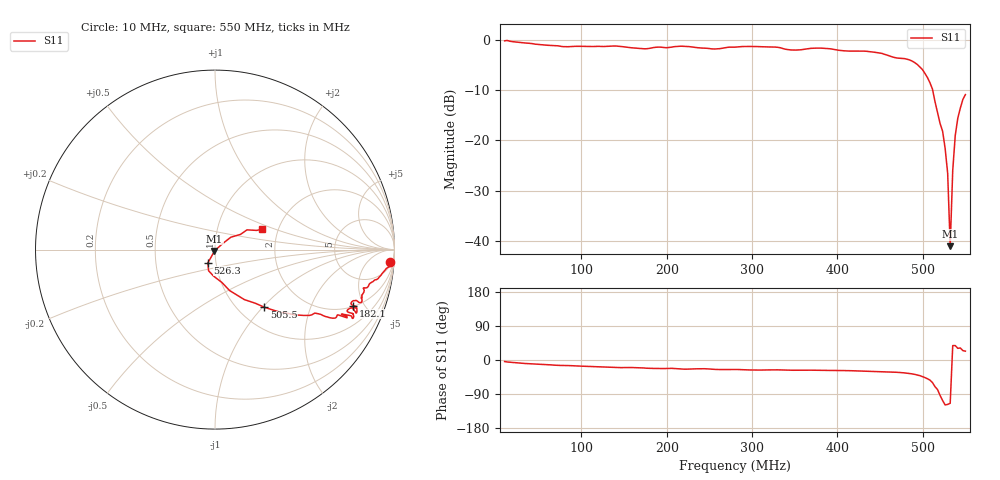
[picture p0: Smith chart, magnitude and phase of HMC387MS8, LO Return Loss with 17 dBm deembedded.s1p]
!Hittite Microwave Corporation
!12 Elizabeth Drive
!Chelmsford, MA 01824
!Tel: 978-250-3343
!Fax: 978-250-3373
!Device: HMC387MS8, 450-500 MHz, GaAs MMIC High IP3 Mixer in 8-lead plastic SMT package
!Misc: LO Return Loss with 17 dBm, Room
# MHZ S MA R 50
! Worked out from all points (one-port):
!   183 points, 10 MHz to 550 MHz, reference 50 ohm
!   lowest |S11| = -41.1 dB at 532.2 MHz (marker M1), VSWR 1.02, Z = 49.6 - j0.799 ohm
!   |S11| at or under -10 dB: 511.6 MHz to end of sweep
!   S11 on the Smith chart (normalised r, x): 10 MHz: 8, -26; 182.1 MHz: 2.06, -4.14; 505.5 MHz: 1.31, -1.02; 526.3 MHz: 0.91, -0.13; 550 MHz: 1.65, +0.40
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10  0.977 -4.0
39.67  0.923 -10.1
78.242  0.856 -14.4
146.484  0.857 -20.1
167.253  0.822 -20.3
182.088  0.83 -22.1
214.725  0.863 -23.6
256.264  0.811 -24.8
280  0.846 -24.9
327.473  0.847 -26.0
348.242  0.791 -27.0
377.912  0.828 -27.3
416.484  0.773 -28.3
452.088  0.733 -30.9
484.725  0.63 -35.6
496.593  0.538 -41.2
505.495  0.422 -49.5
511.429  0.323 -59.6
514.396  0.242 -70.4
523.297  0.123 -106.9
526.264  0.083 -118.6
529.231  0.047 -117.2
532.198  0.008826 -114.2
535.165  0.05 38.0
538.132  0.112 38.0
541.099  0.166 30.8
547.033  0.255 24.8
550  0.285 23.3
